(* Logix 5000 AddOnInstructionDefinition export Banner_S15S_TH_Param_v4; software revision 33.03 *)

TYPE Banner_Direct_Parameters_v4 :
STRUCT
   Master_Cycle_Time : INT;
   Min_Cycle_Time : INT;
   M_Sequence_Capability : INT;
   IO_Link_Version_ID : INT;
   Process_Data_Input_Length : INT;
   Process_Data_Output_Length : INT;
   Combined_Vendor_ID : DINT;   // IO-Link Vendor ID
   Vendor_ID1 : INT;
   Vendor_ID2 : INT;
   Combined_Device_ID : DINT;   // IO-Link Device ID
   Device_ID1 : INT;
   Device_ID2 : INT;
   Device_ID3 : INT;
END_STRUCT
END_TYPE

TYPE Banner_IOL_Port_v4 :   // UDT that has all of the data items necessary to communicate with a specific Port on a IO-Link Master
STRUCT
   Port_Controlled : INT;   // Each bit represents a port on an IO-Link Master. Set to 1 to tell AOI to control that port.
   Port_Activate : INT;   // Each bit represents a port on an IO-Link Master. When ON that port will process any commands in queue.
   Port_Read : INT;   // Each bit represents a port on an IO-Link Master. Used to determine when device AOI has requested a Read command.
   Port_Write : INT;   // Each bit represents a port on an IO-Link Master. Used to determine when device AOI has requested a Write command.
   Port_RW_Complete : INT;   // Each bit represents a port on an IO-Link Master. Tells device AOI that Read or Write request has been completed.
   Port_Device_Read : INT;
   Data_Transfer : SINT[190];   // Array to transfer data from IO-Master to device AOIs.
END_STRUCT
END_TYPE

TYPE Banner_S15S_TH_Alarm_Configuration_v4 :
STRUCT
   Temp_Low_Threshold : REAL;
   Temp_High_Threshold : REAL;
   Relative_Humidity_Low_Threshold : REAL;
   Relative_Humidity_High_Threshold : REAL;
   Dew_Point_Low_Threshold : REAL;
   Dew_Point_High_Threshold : REAL;
   Temp_On_Delay : REAL;
   Temp_Off_Delay : REAL;
   Relative_Humidity_On_Delay : REAL;
   Relative_Humidity_Off_Delay : REAL;
   Dew_Point_On_Delay : REAL;
   Dew_Point_Off_Delay : REAL;
END_STRUCT
END_TYPE

TYPE Banner_S15S_TH_Alarm_Counters_v4 :
STRUCT
   Temp_Low_Counter : DINT;
   Temp_High_Counter : DINT;
   Relative_Humidity_Low_Counter : DINT;
   Relative_Humidity_High_Counter : DINT;
   Dew_Point_Low_Counter : DINT;
   Dew_Point_High_Counter : DINT;
END_STRUCT
END_TYPE

TYPE Banner_S15S_TH_RD_v4 :   // UDT that stores the Read Data for a S15S-TH-KQ.
STRUCT
   Direct : Banner_Direct_Parameters_v4;
   Serial_Number : STRING;
   All_Time_Run_Time : DINT;   // 0 to 2 Billion. 1/4 hr increments.
END_STRUCT
END_TYPE

TYPE Banner_S15S_TH_v4 :   // All of the parameters for a S15S-TH-KQ.
STRUCT
   Initial_Global_Read : BOOL;   // Determines if all of the IO-Link data has been read into the PLC yet
   Command : INT;   // Value placed in here will activate a read or write to a specifc IO-Link Index
   Read : Banner_S15S_TH_RD_v4;   // Read Only Data
   Write : Banner_S15S_TH_WD_v4;   // Write Data
   Reset : BOOL;   // Resets AOI. This will force a complete parameter read of the sensor.
END_STRUCT
END_TYPE

TYPE Banner_S15S_TH_WD_v4 :   // UDT that stores the Write Data for a S15S-TH-KQ.
STRUCT
   System_Command : INT;   // See IODD file for list of commands that can be activated via the System Command interface
   Parameter_Access_Lock : SINT;   // Write access to all parameters is prohibited while value is 1. Only this parameter can be adjusted when value is 1.
   Data_Storage_Lock : SINT;   // Automatic data storage is disabled when this value is equal to 1. Read access is not affected.
   Local_Parameterization_Lock : SINT;   // Parameterization via local control elements on device is disabled.
   Local_User_Interface_Lock : SINT;   // Operation of local user interface is disabled.
   Resettable_Run_Time_Counter : DINT;   // 0 to 2 Billion. 1/4 hr increments.
   Alarm_Config : Banner_S15S_TH_Alarm_Configuration_v4;
   Alarm_Counters : Banner_S15S_TH_Alarm_Counters_v4;
   Process_Data_Mode : INT;   // 1=Smart Sensor Profile, Fahrenheit, 2=Smart Sensor Profile, Celsius, 3=Floating Point, Fahrenheit, 4=Floating Point, Celsius
   Output_Config : INT;   // 0=BannerBus,1=Discrete Output
END_STRUCT
END_TYPE

ADD_ON_INSTRUCTION Banner_S15S_TH_Float_In_v4   (* revision 4.0 *)
// AOI the orientates the bytes for a floating point value.
VAR_IN_OUT
   Float : REAL; {required}
END_VAR
VAR_INPUT
   Sint0 : SINT; {required}
   Sint1 : SINT; {required}
   Sint2 : SINT; {required}
   Sint3 : SINT; {required}
END_VAR
VAR
   Temp_Byte : SINT[4]; {access None}
END_VAR

ROUTINE Logic   (* ladder *)
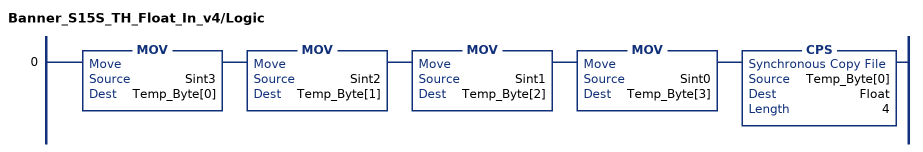
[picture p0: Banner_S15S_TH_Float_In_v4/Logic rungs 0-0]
   0: MOV(Sint3,Temp_Byte[0])MOV(Sint2,Temp_Byte[1])MOV(Sint1,Temp_Byte[2])MOV(Sint0,Temp_Byte[3])CPS(Temp_Byte[0],Float,4);
END_ROUTINE
END_ADD_ON_INSTRUCTION

ADD_ON_INSTRUCTION Banner_S15S_TH_Float_Out_v4   (* revision 4.0 *)
// AOI the orientates the bytes for a floating point value.
VAR_INPUT
   Float : REAL; {required}
END_VAR
VAR_IN_OUT
   Sint0 : SINT; {required}
   Sint1 : SINT; {required}
   Sint2 : SINT; {required}
   Sint3 : SINT; {required}
END_VAR
VAR
   Temp_Byte : SINT[4]; {access None}
END_VAR

ROUTINE Logic   (* ladder *)
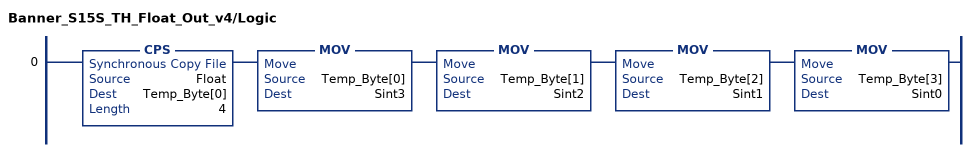
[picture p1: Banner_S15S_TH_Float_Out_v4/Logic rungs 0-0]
   0: CPS(Float,Temp_Byte[0],4)MOV(Temp_Byte[0],Sint3)MOV(Temp_Byte[1],Sint2)MOV(Temp_Byte[2],Sint1)MOV(Temp_Byte[3],Sint0);
END_ROUTINE
END_ADD_ON_INSTRUCTION

ADD_ON_INSTRUCTION Banner_S15S_TH_Param_v4   (* revision 4.0, vendor Banner Engineering *)
// AOI to read and write parameter data to an IO-Link S15S-TH-KQ.
VAR_IN_OUT
   S15STH : Banner_S15S_TH_v4; {required}
   Port_Data : Banner_IOL_Port_v4; {required}
END_VAR
VAR_INPUT
   Port : DINT; {required}
END_VAR
VAR
   Local_Control : DINT; {access None}
   Global_Read_Command_Value : INT; {access None}
   Global_Write_Command_Value : INT; {access None}
   Command_Being_Processed : BOOL; {access None}
   Update_Archive : BOOL; {access None}
   Index_Write_Inprocess : INT; {access None}
   Index_Write_Control : INT; {access None}
   Inprocess_Index : DINT; {access None}
   AOI_Out_Status : Banner_S15S_TH_Float_Out_v4[12]; {access None}
   AOI_In_Status : Banner_S15S_TH_Float_In_v4[12]; {access None}
END_VAR

ROUTINE Logic   (* ladder *)
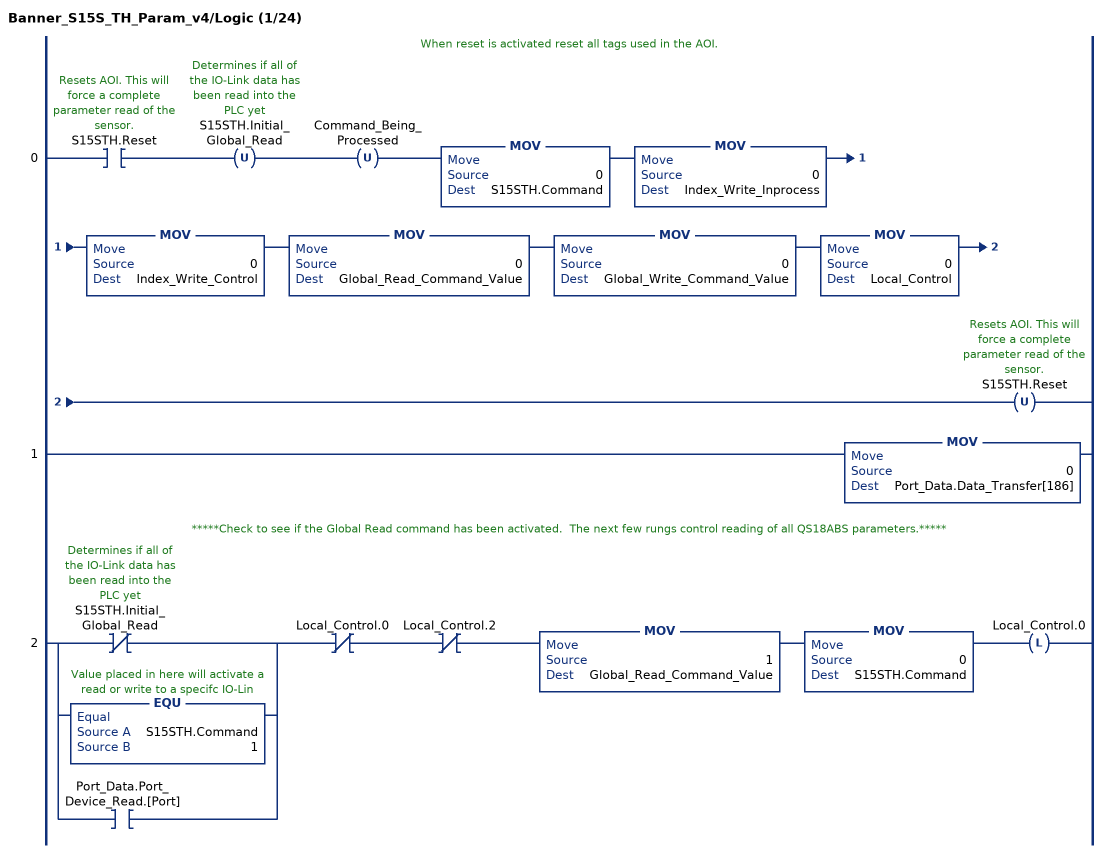
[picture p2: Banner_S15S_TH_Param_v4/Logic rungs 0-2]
   // When reset is activated reset all tags used in the AOI.
   0: XIC(S15STH.Reset)OTU(S15STH.Initial_Global_Read)OTU(Command_Being_Processed)MOV(0,S15STH.Command)MOV(0,Index_Write_Inprocess)MOV(0,Index_Write_Control)MOV(0,Global_Read_Command_Value)MOV(0,Global_Write_Command_Value)MOV(0,Local_Control)OTU(S15STH.Reset);
   1: MOV(0,Port_Data.Data_Transfer[186]);
   // *****Check to see if the Global Read command has been activated.  The next few rungs control reading of all QS18ABS parameters.*****
   2: [XIO(S15STH.Initial_Global_Read) ,EQU(S15STH.Command,1) ,XIC(Port_Data.Port_Device_Read.[Port]) ]XIO(Local_Control.0)XIO(Local_Control.2)MOV(1,Global_Read_Command_Value)MOV(0,S15STH.Command)OTL(Local_Control.0);
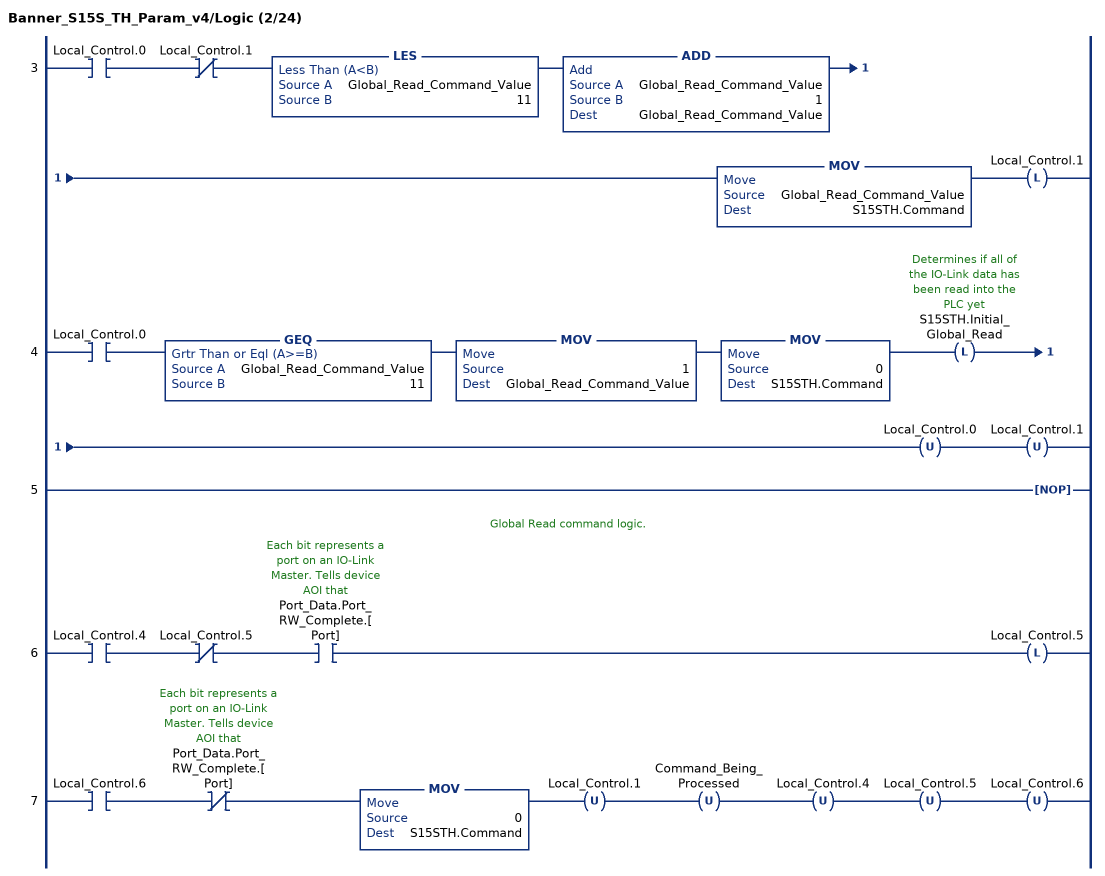
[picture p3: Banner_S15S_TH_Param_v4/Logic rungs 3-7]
   3: XIC(Local_Control.0)XIO(Local_Control.1)LES(Global_Read_Command_Value,11)ADD(Global_Read_Command_Value,1,Global_Read_Command_Value)MOV(Global_Read_Command_Value,S15STH.Command)OTL(Local_Control.1);
   4: XIC(Local_Control.0)GEQ(Global_Read_Command_Value,11)MOV(1,Global_Read_Command_Value)MOV(0,S15STH.Command)OTL(S15STH.Initial_Global_Read)OTU(Local_Control.0)OTU(Local_Control.1);
   5: NOP();
   // Global Read command logic.
   6: XIC(Local_Control.4)XIO(Local_Control.5)XIC(Port_Data.Port_RW_Complete.[Port])OTL(Local_Control.5);
   7: XIC(Local_Control.6)XIO(Port_Data.Port_RW_Complete.[Port])MOV(0,S15STH.Command)OTU(Local_Control.1)OTU(Command_Being_Processed)OTU(Local_Control.4)OTU(Local_Control.5)OTU(Local_Control.6);
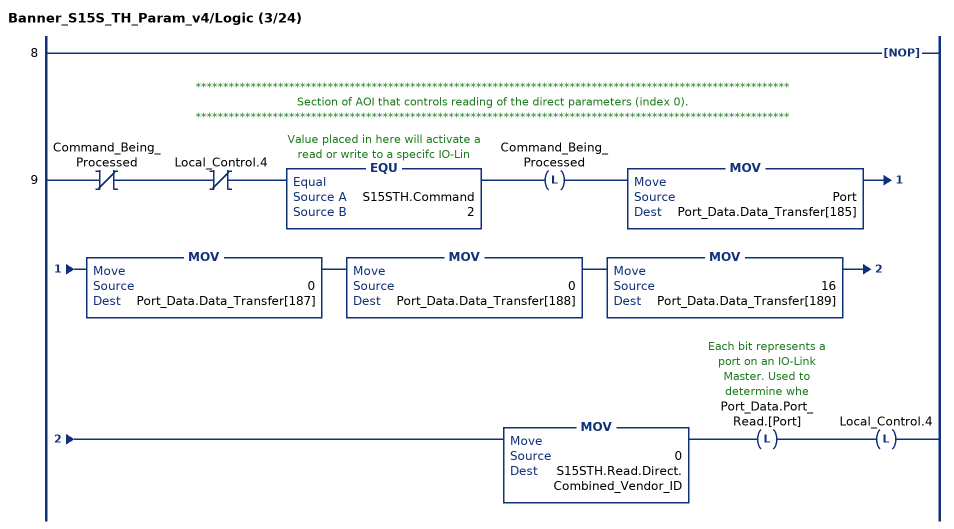
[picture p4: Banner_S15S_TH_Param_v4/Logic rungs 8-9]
   8: NOP();
   // ************************************************************************************************************
   // Section of AOI that controls reading of the direct parameters (index 0).
   // ************************************************************************************************************
   9: XIO(Command_Being_Processed)XIO(Local_Control.4)EQU(S15STH.Command,2)OTL(Command_Being_Processed)MOV(Port,Port_Data.Data_Transfer[185])MOV(0,Port_Data.Data_Transfer[187])MOV(0,Port_Data.Data_Transfer[188])MOV(16,Port_Data.Data_Transfer[189])MOV(0,S15STH.Read.Direct.Combined_Vendor_ID)OTL(Port_Data.Port_Read.[Port])OTL(Local_Control.4);
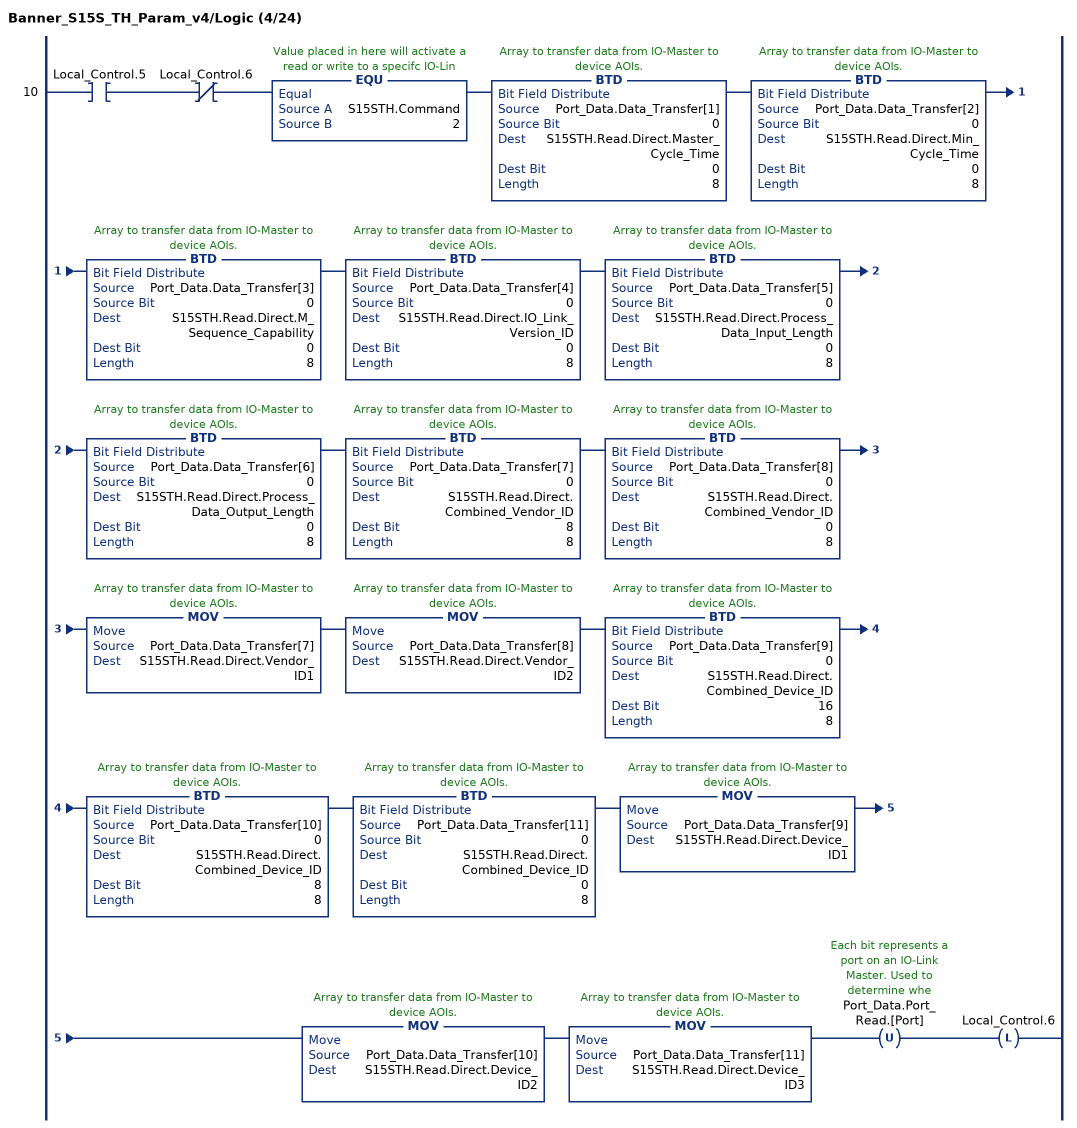
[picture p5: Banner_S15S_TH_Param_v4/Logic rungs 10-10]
   10: XIC(Local_Control.5)XIO(Local_Control.6)EQU(S15STH.Command,2)BTD(Port_Data.Data_Transfer[1],0,S15STH.Read.Direct.Master_Cycle_Time,0,8)BTD(Port_Data.Data_Transfer[2],0,S15STH.Read.Direct.Min_Cycle_Time,0,8)BTD(Port_Data.Data_Transfer[3],0,S15STH.Read.Direct.M_Sequence_Capability,0,8)BTD(Port_Data.Data_Transfer[4],0,S15STH.Read.Direct.IO_Link_Version_ID,0,8)BTD(Port_Data.Data_Transfer[5],0,S15STH.Read.Direct.Process_Data_Input_Length,0,8)BTD(Port_Data.Data_Transfer[6],0,S15STH.Read.Direct.Process_Data_Output_Length,0,8)BTD(Port_Data.Data_Transfer[7],0,S15STH.Read.Direct.Combined_Vendor_ID,8,8)BTD(Port_Data.Data_Transfer[8],0,S15STH.Read.Direct.Combined_Vendor_ID,0,8)MOV(Port_Data.Data_Transfer[7],S15STH.Read.Direct.Vendor_ID1)MOV(Port_Data.Data_Transfer[8],S15STH.Read.Direct.Vendor_ID2)BTD(Port_Data.Data_Transfer[9],0,S15STH.Read.Direct.Combined_Device_ID,16,8)BTD(Port_Data.Data_Transfer[10],0,S15STH.Read.Direct.Combined_Device_ID,8,8)BTD(Port_Data.Data_Transfer[11],0,S15STH.Read.Direct.Combined_Device_ID,0,8)MOV(Port_Data.Data_Transfer[9],S15STH.Read.Direct.Device_ID1)MOV(Port_Data.Data_Transfer[10],S15STH.Read.Direct.Device_ID2)MOV(Port_Data.Data_Transfer[11],S15STH.Read.Direct.Device_ID3)OTU(Port_Data.Port_Read.[Port])OTL(Local_Control.6);
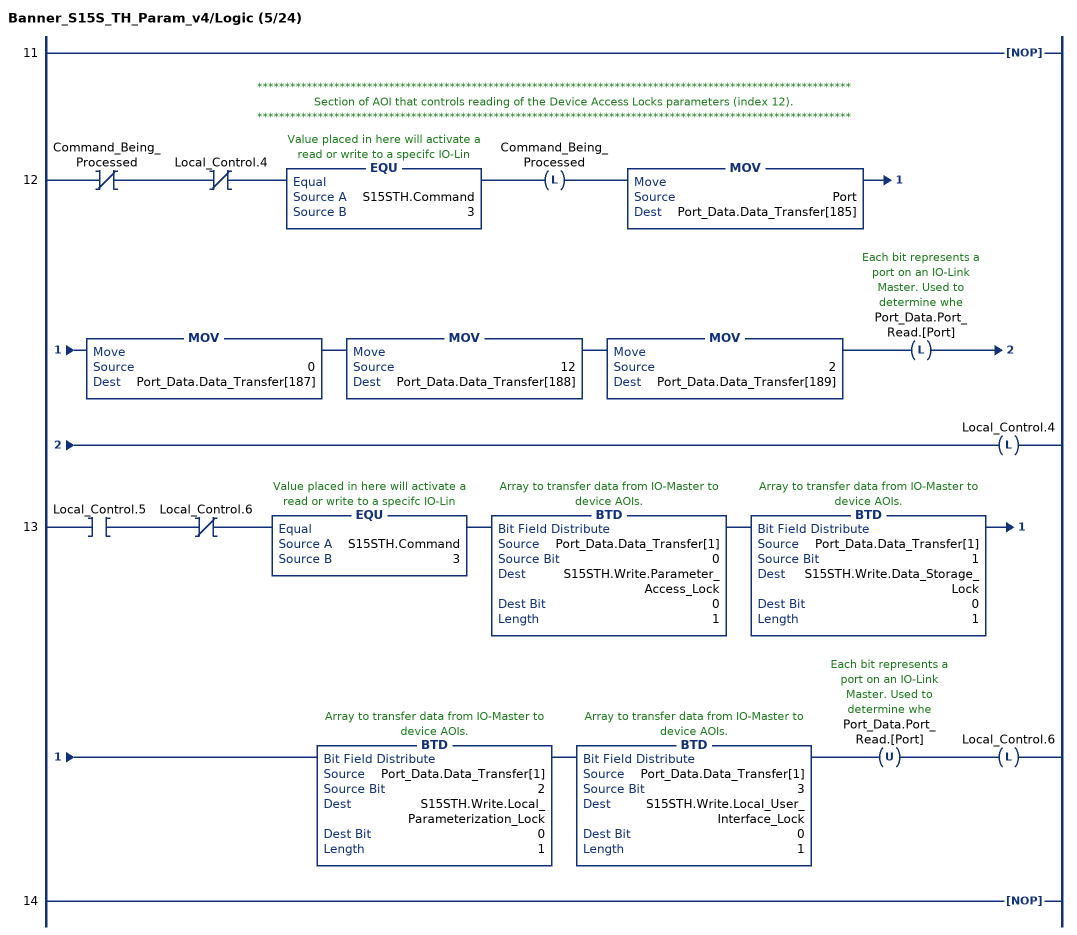
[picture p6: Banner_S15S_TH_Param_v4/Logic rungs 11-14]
   11: NOP();
   // ************************************************************************************************************
   // Section of AOI that controls reading of the Device Access Locks parameters (index 12).
   // ************************************************************************************************************
   12: XIO(Command_Being_Processed)XIO(Local_Control.4)EQU(S15STH.Command,3)OTL(Command_Being_Processed)MOV(Port,Port_Data.Data_Transfer[185])MOV(0,Port_Data.Data_Transfer[187])MOV(12,Port_Data.Data_Transfer[188])MOV(2,Port_Data.Data_Transfer[189])OTL(Port_Data.Port_Read.[Port])OTL(Local_Control.4);
   13: XIC(Local_Control.5)XIO(Local_Control.6)EQU(S15STH.Command,3)BTD(Port_Data.Data_Transfer[1],0,S15STH.Write.Parameter_Access_Lock,0,1)BTD(Port_Data.Data_Transfer[1],1,S15STH.Write.Data_Storage_Lock,0,1)BTD(Port_Data.Data_Transfer[1],2,S15STH.Write.Local_Parameterization_Lock,0,1)BTD(Port_Data.Data_Transfer[1],3,S15STH.Write.Local_User_Interface_Lock,0,1)OTU(Port_Data.Port_Read.[Port])OTL(Local_Control.6);
   14: NOP();
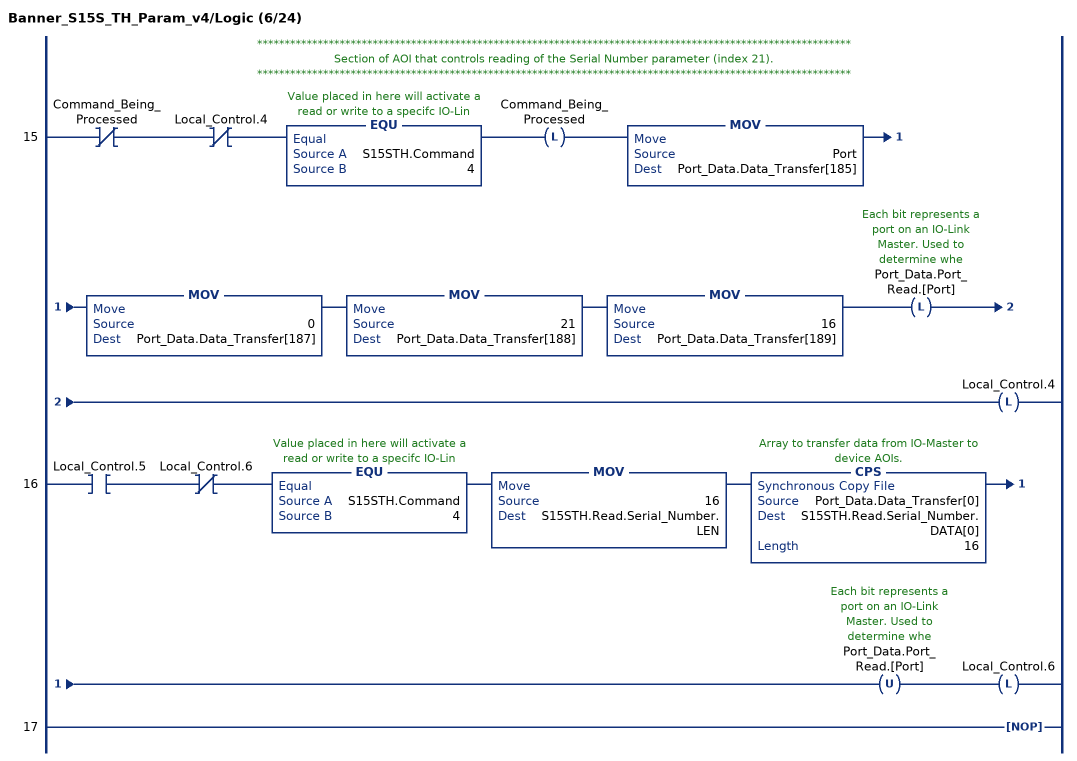
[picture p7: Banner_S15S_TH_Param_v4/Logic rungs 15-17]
   // ************************************************************************************************************
   // Section of AOI that controls reading of the Serial Number parameter (index 21).
   // ************************************************************************************************************
   15: XIO(Command_Being_Processed)XIO(Local_Control.4)EQU(S15STH.Command,4)OTL(Command_Being_Processed)MOV(Port,Port_Data.Data_Transfer[185])MOV(0,Port_Data.Data_Transfer[187])MOV(21,Port_Data.Data_Transfer[188])MOV(16,Port_Data.Data_Transfer[189])OTL(Port_Data.Port_Read.[Port])OTL(Local_Control.4);
   16: XIC(Local_Control.5)XIO(Local_Control.6)EQU(S15STH.Command,4)MOV(16,S15STH.Read.Serial_Number.LEN)CPS(Port_Data.Data_Transfer[0],S15STH.Read.Serial_Number.DATA[0],16)OTU(Port_Data.Port_Read.[Port])OTL(Local_Control.6);
   17: NOP();
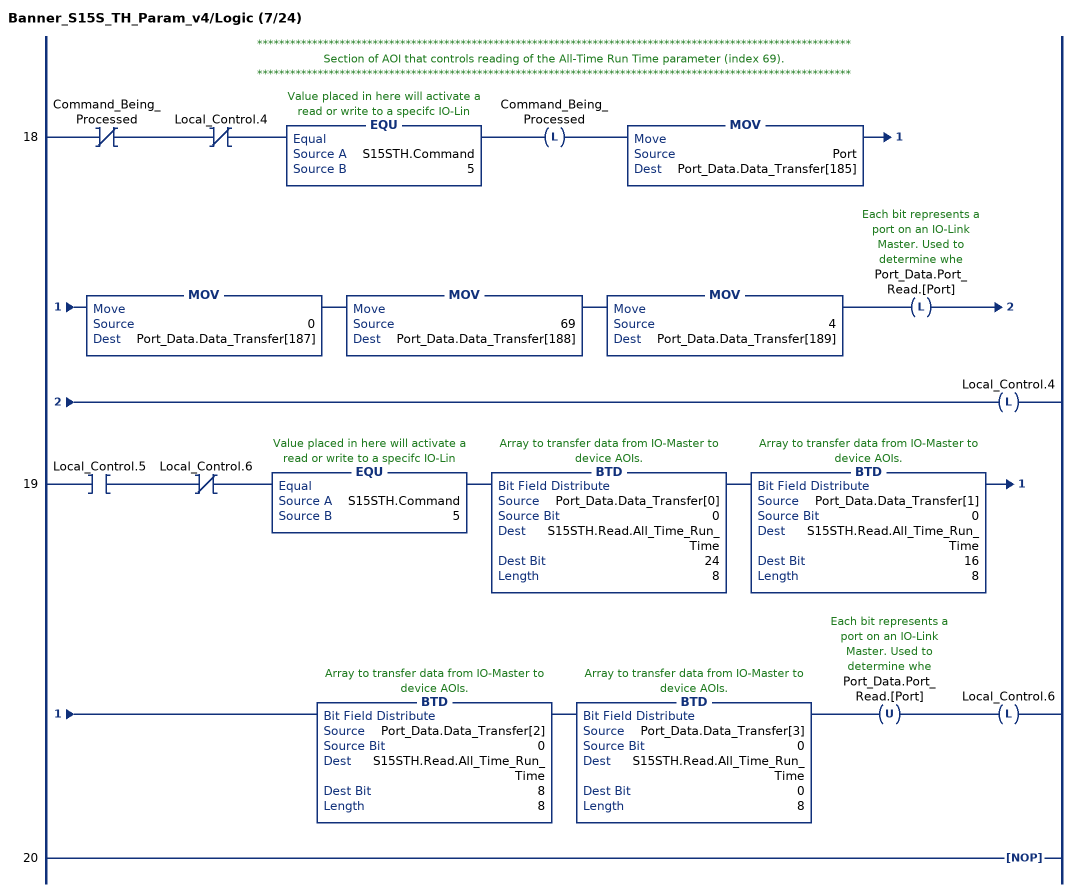
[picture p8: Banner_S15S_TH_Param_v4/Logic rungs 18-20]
   // ************************************************************************************************************
   // Section of AOI that controls reading of the All-Time Run Time parameter (index 69).
   // ************************************************************************************************************
   18: XIO(Command_Being_Processed)XIO(Local_Control.4)EQU(S15STH.Command,5)OTL(Command_Being_Processed)MOV(Port,Port_Data.Data_Transfer[185])MOV(0,Port_Data.Data_Transfer[187])MOV(69,Port_Data.Data_Transfer[188])MOV(4,Port_Data.Data_Transfer[189])OTL(Port_Data.Port_Read.[Port])OTL(Local_Control.4);
   19: XIC(Local_Control.5)XIO(Local_Control.6)EQU(S15STH.Command,5)BTD(Port_Data.Data_Transfer[0],0,S15STH.Read.All_Time_Run_Time,24,8)BTD(Port_Data.Data_Transfer[1],0,S15STH.Read.All_Time_Run_Time,16,8)BTD(Port_Data.Data_Transfer[2],0,S15STH.Read.All_Time_Run_Time,8,8)BTD(Port_Data.Data_Transfer[3],0,S15STH.Read.All_Time_Run_Time,0,8)OTU(Port_Data.Port_Read.[Port])OTL(Local_Control.6);
   20: NOP();
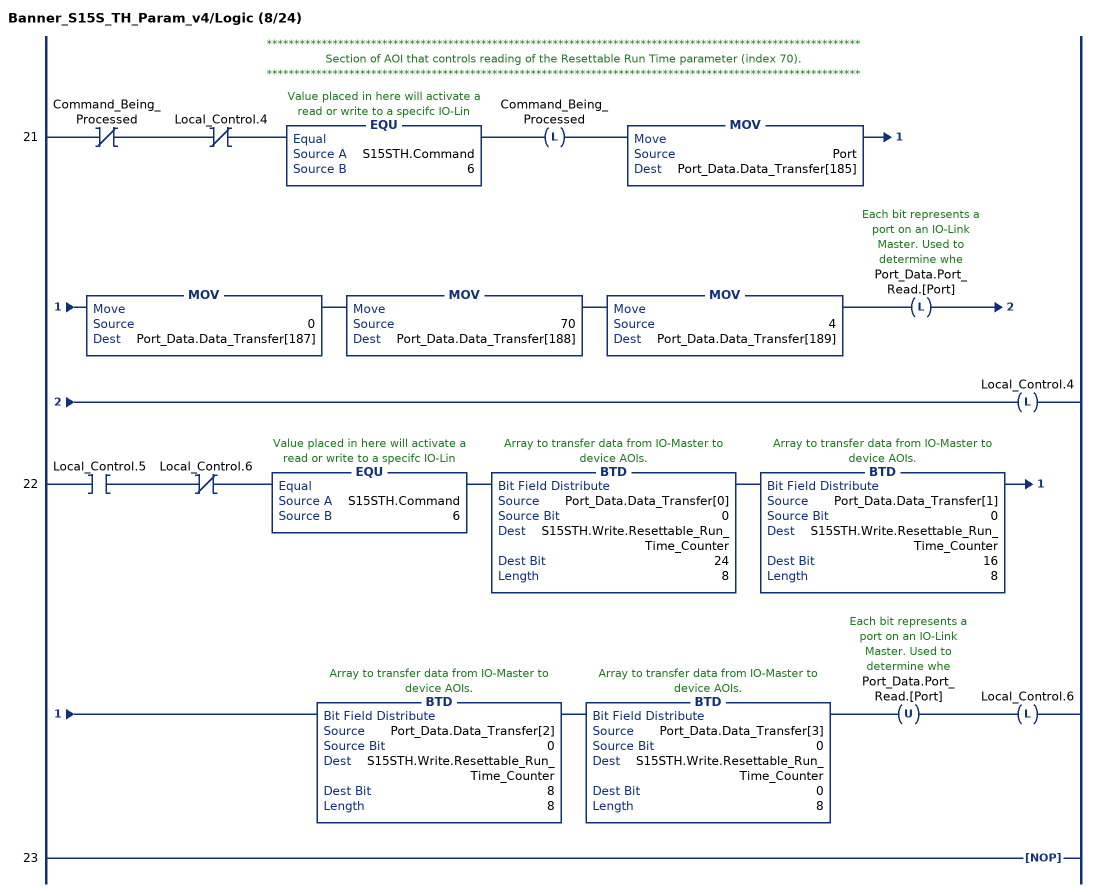
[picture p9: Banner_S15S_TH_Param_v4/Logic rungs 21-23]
   // ************************************************************************************************************
   // Section of AOI that controls reading of the Resettable Run Time parameter (index 70).
   // ************************************************************************************************************
   21: XIO(Command_Being_Processed)XIO(Local_Control.4)EQU(S15STH.Command,6)OTL(Command_Being_Processed)MOV(Port,Port_Data.Data_Transfer[185])MOV(0,Port_Data.Data_Transfer[187])MOV(70,Port_Data.Data_Transfer[188])MOV(4,Port_Data.Data_Transfer[189])OTL(Port_Data.Port_Read.[Port])OTL(Local_Control.4);
   22: XIC(Local_Control.5)XIO(Local_Control.6)EQU(S15STH.Command,6)BTD(Port_Data.Data_Transfer[0],0,S15STH.Write.Resettable_Run_Time_Counter,24,8)BTD(Port_Data.Data_Transfer[1],0,S15STH.Write.Resettable_Run_Time_Counter,16,8)BTD(Port_Data.Data_Transfer[2],0,S15STH.Write.Resettable_Run_Time_Counter,8,8)BTD(Port_Data.Data_Transfer[3],0,S15STH.Write.Resettable_Run_Time_Counter,0,8)OTU(Port_Data.Port_Read.[Port])OTL(Local_Control.6);
   23: NOP();
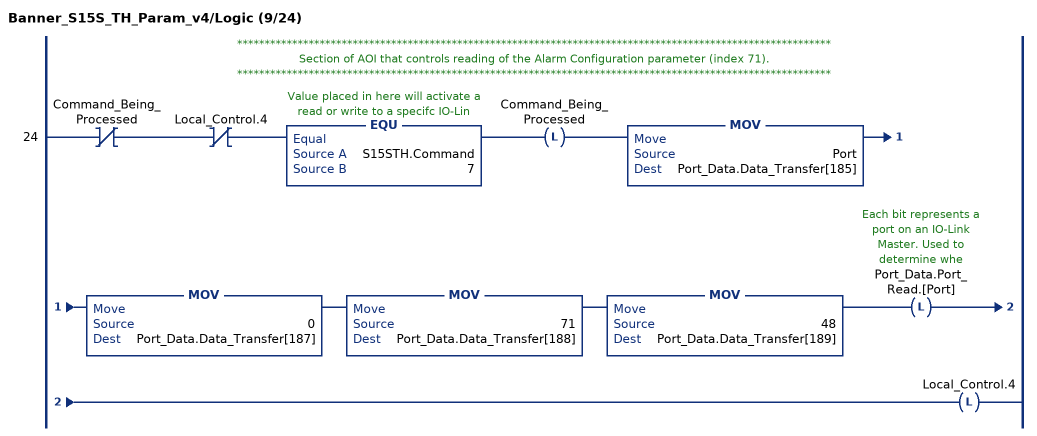
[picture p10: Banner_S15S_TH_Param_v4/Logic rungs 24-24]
   // ************************************************************************************************************
   // Section of AOI that controls reading of the Alarm Configuration parameter (index 71).
   // ************************************************************************************************************
   24: XIO(Command_Being_Processed)XIO(Local_Control.4)EQU(S15STH.Command,7)OTL(Command_Being_Processed)MOV(Port,Port_Data.Data_Transfer[185])MOV(0,Port_Data.Data_Transfer[187])MOV(71,Port_Data.Data_Transfer[188])MOV(48,Port_Data.Data_Transfer[189])OTL(Port_Data.Port_Read.[Port])OTL(Local_Control.4);
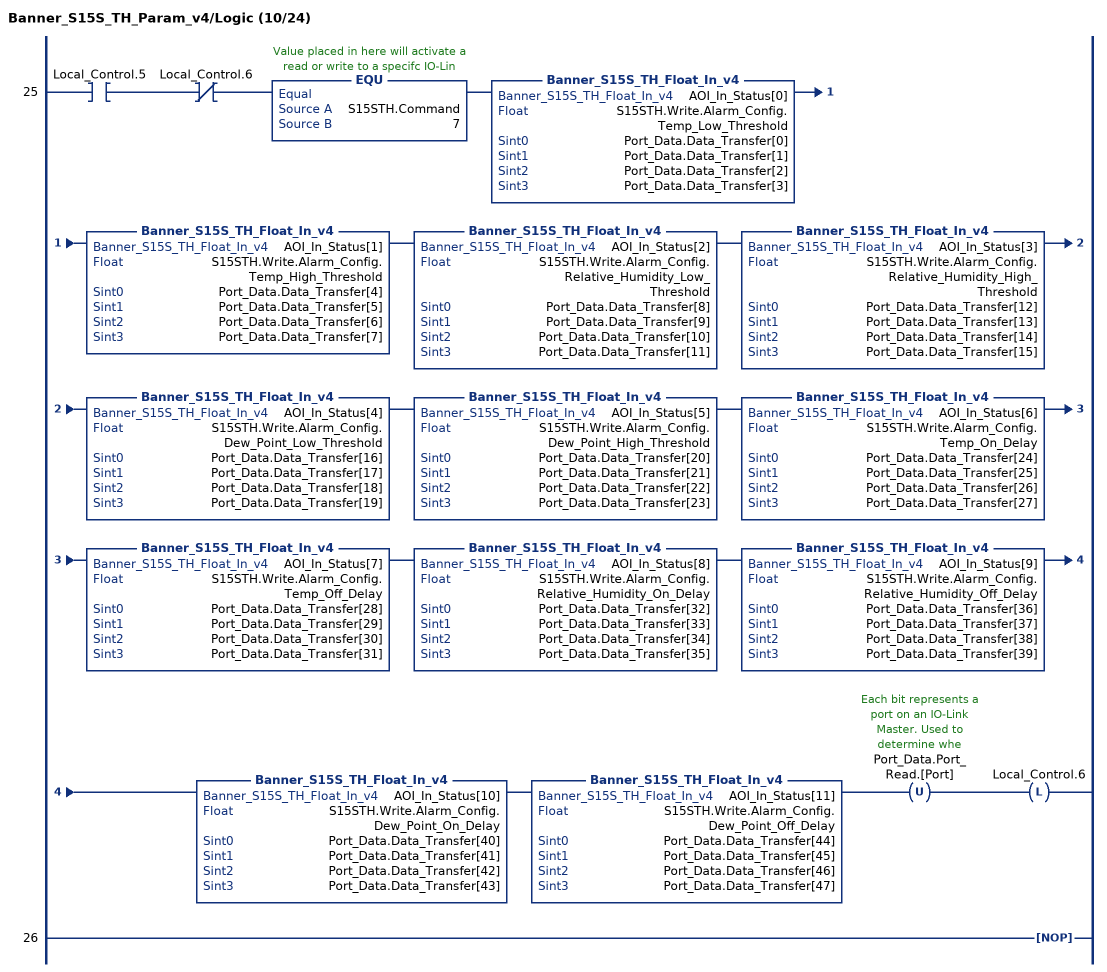
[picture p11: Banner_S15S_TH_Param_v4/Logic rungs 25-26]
   25: XIC(Local_Control.5)XIO(Local_Control.6)EQU(S15STH.Command,7)Banner_S15S_TH_Float_In_v4(AOI_In_Status[0],S15STH.Write.Alarm_Config.Temp_Low_Threshold,Port_Data.Data_Transfer[0],Port_Data.Data_Transfer[1],Port_Data.Data_Transfer[2],Port_Data.Data_Transfer[3])Banner_S15S_TH_Float_In_v4(AOI_In_Status[1],S15STH.Write.Alarm_Config.Temp_High_Threshold,Port_Data.Data_Transfer[4],Port_Data.Data_Transfer[5],Port_Data.Data_Transfer[6],Port_Data.Data_Transfer[7])Banner_S15S_TH_Float_In_v4(AOI_In_Status[2],S15STH.Write.Alarm_Config.Relative_Humidity_Low_Threshold,Port_Data.Data_Transfer[8],Port_Data.Data_Transfer[9],Port_Data.Data_Transfer[10],Port_Data.Data_Transfer[11])Banner_S15S_TH_Float_In_v4(AOI_In_Status[3],S15STH.Write.Alarm_Config.Relative_Humidity_High_Threshold,Port_Data.Data_Transfer[12],Port_Data.Data_Transfer[13],Port_Data.Data_Transfer[14],Port_Data.Data_Transfer[15])Banner_S15S_TH_Float_In_v4(AOI_In_Status[4],S15STH.Write.Alarm_Config.Dew_Point_Low_Threshold,Port_Data.Data_Transfer[16],Port_Data.Data_Transfer[17],Port_Data.Data_Transfer[18],Port_Data.Data_Transfer[19])Banner_S15S_TH_Float_In_v4(AOI_In_Status[5],S15STH.Write.Alarm_Config.Dew_Point_High_Threshold,Port_Data.Data_Transfer[20],Port_Data.Data_Transfer[21],Port_Data.Data_Transfer[22],Port_Data.Data_Transfer[23])Banner_S15S_TH_Float_In_v4(AOI_In_Status[6],S15STH.Write.Alarm_Config.Temp_On_Delay,Port_Data.Data_Transfer[24],Port_Data.Data_Transfer[25],Port_Data.Data_Transfer[26],Port_Data.Data_Transfer[27])Banner_S15S_TH_Float_In_v4(AOI_In_Status[7],S15STH.Write.Alarm_Config.Temp_Off_Delay,Port_Data.Data_Transfer[28],Port_Data.Data_Transfer[29],Port_Data.Data_Transfer[30],Port_Data.Data_Transfer[31])Banner_S15S_TH_Float_In_v4(AOI_In_Status[8],S15STH.Write.Alarm_Config.Relative_Humidity_On_Delay,Port_Data.Data_Transfer[32],Port_Data.Data_Transfer[33],Port_Data.Data_Transfer[34],Port_Data.Data_Transfer[35])Banner_S15S_TH_Float_In_v4(AOI_In_Status[9],S15STH.Write.Alarm_Config.Relative_Humidity_Off_Delay,Port_Data.Data_Transfer[36],Port_Data.Data_Transfer[37],Port_Data.Data_Transfer[38],Port_Data.Data_Transfer[39])Banner_S15S_TH_Float_In_v4(AOI_In_Status[10],S15STH.Write.Alarm_Config.Dew_Point_On_Delay,Port_Data.Data_Transfer[40],Port_Data.Data_Transfer[41],Port_Data.Data_Transfer[42],Port_Data.Data_Transfer[43])Banner_S15S_TH_Float_In_v4(AOI_In_Status[11],S15STH.Write.Alarm_Config.Dew_Point_Off_Delay,Port_Data.Data_Transfer[44],Port_Data.Data_Transfer[45],Port_Data.Data_Transfer[46],Port_Data.Data_Transfer[47])OTU(Port_Data.Port_Read.[Port])OTL(Local_Control.6);
   26: NOP();
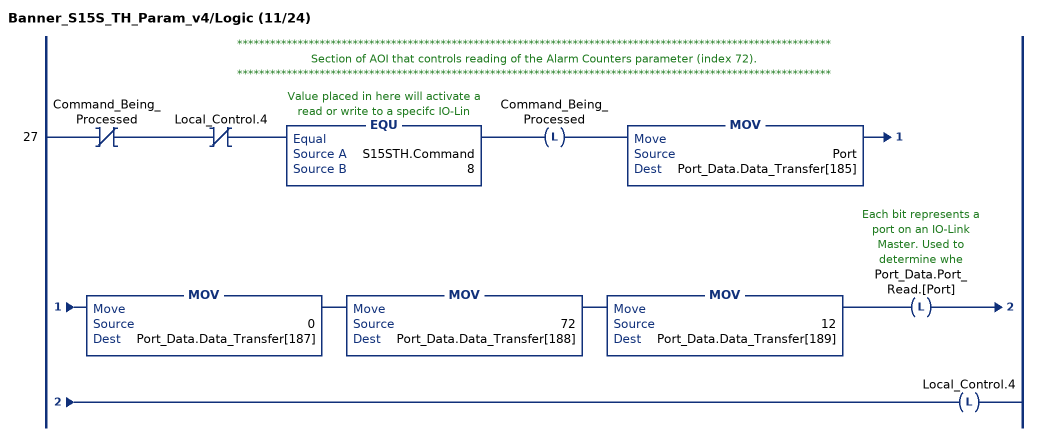
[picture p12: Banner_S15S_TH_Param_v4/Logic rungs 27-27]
   // ************************************************************************************************************
   // Section of AOI that controls reading of the Alarm Counters parameter (index 72).
   // ************************************************************************************************************
   27: XIO(Command_Being_Processed)XIO(Local_Control.4)EQU(S15STH.Command,8)OTL(Command_Being_Processed)MOV(Port,Port_Data.Data_Transfer[185])MOV(0,Port_Data.Data_Transfer[187])MOV(72,Port_Data.Data_Transfer[188])MOV(12,Port_Data.Data_Transfer[189])OTL(Port_Data.Port_Read.[Port])OTL(Local_Control.4);
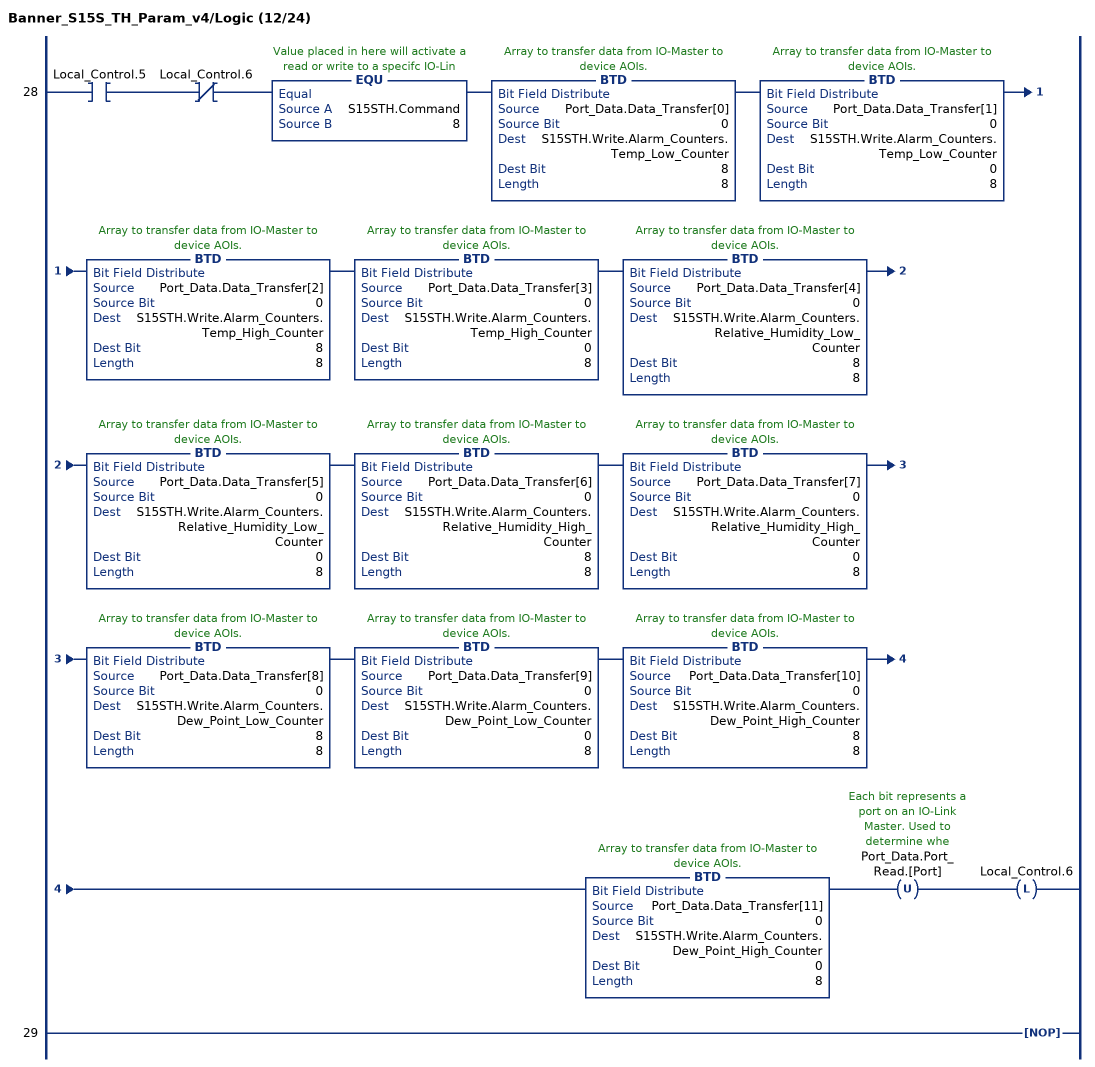
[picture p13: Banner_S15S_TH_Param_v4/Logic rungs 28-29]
   28: XIC(Local_Control.5)XIO(Local_Control.6)EQU(S15STH.Command,8)BTD(Port_Data.Data_Transfer[0],0,S15STH.Write.Alarm_Counters.Temp_Low_Counter,8,8)BTD(Port_Data.Data_Transfer[1],0,S15STH.Write.Alarm_Counters.Temp_Low_Counter,0,8)BTD(Port_Data.Data_Transfer[2],0,S15STH.Write.Alarm_Counters.Temp_High_Counter,8,8)BTD(Port_Data.Data_Transfer[3],0,S15STH.Write.Alarm_Counters.Temp_High_Counter,0,8)BTD(Port_Data.Data_Transfer[4],0,S15STH.Write.Alarm_Counters.Relative_Humidity_Low_Counter,8,8)BTD(Port_Data.Data_Transfer[5],0,S15STH.Write.Alarm_Counters.Relative_Humidity_Low_Counter,0,8)BTD(Port_Data.Data_Transfer[6],0,S15STH.Write.Alarm_Counters.Relative_Humidity_High_Counter,8,8)BTD(Port_Data.Data_Transfer[7],0,S15STH.Write.Alarm_Counters.Relative_Humidity_High_Counter,0,8)BTD(Port_Data.Data_Transfer[8],0,S15STH.Write.Alarm_Counters.Dew_Point_Low_Counter,8,8)BTD(Port_Data.Data_Transfer[9],0,S15STH.Write.Alarm_Counters.Dew_Point_Low_Counter,0,8)BTD(Port_Data.Data_Transfer[10],0,S15STH.Write.Alarm_Counters.Dew_Point_High_Counter,8,8)BTD(Port_Data.Data_Transfer[11],0,S15STH.Write.Alarm_Counters.Dew_Point_High_Counter,0,8)OTU(Port_Data.Port_Read.[Port])OTL(Local_Control.6);
   29: NOP();
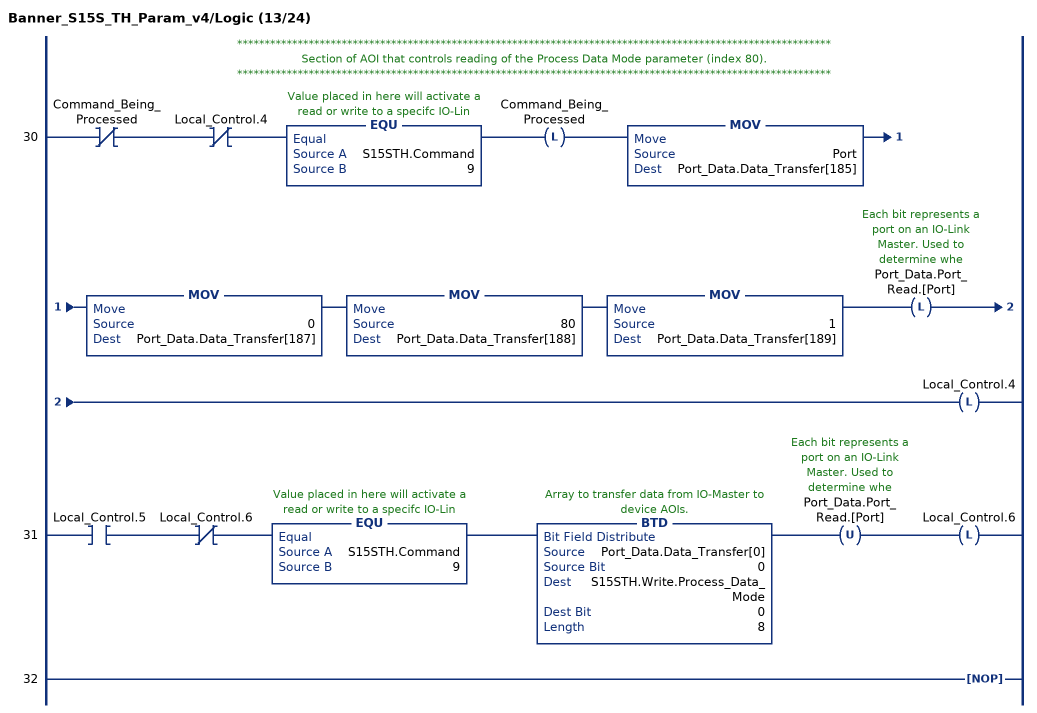
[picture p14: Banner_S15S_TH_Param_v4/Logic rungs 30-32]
   // ************************************************************************************************************
   // Section of AOI that controls reading of the Process Data Mode parameter (index 80).
   // ************************************************************************************************************
   30: XIO(Command_Being_Processed)XIO(Local_Control.4)EQU(S15STH.Command,9)OTL(Command_Being_Processed)MOV(Port,Port_Data.Data_Transfer[185])MOV(0,Port_Data.Data_Transfer[187])MOV(80,Port_Data.Data_Transfer[188])MOV(1,Port_Data.Data_Transfer[189])OTL(Port_Data.Port_Read.[Port])OTL(Local_Control.4);
   31: XIC(Local_Control.5)XIO(Local_Control.6)EQU(S15STH.Command,9)BTD(Port_Data.Data_Transfer[0],0,S15STH.Write.Process_Data_Mode,0,8)OTU(Port_Data.Port_Read.[Port])OTL(Local_Control.6);
   32: NOP();
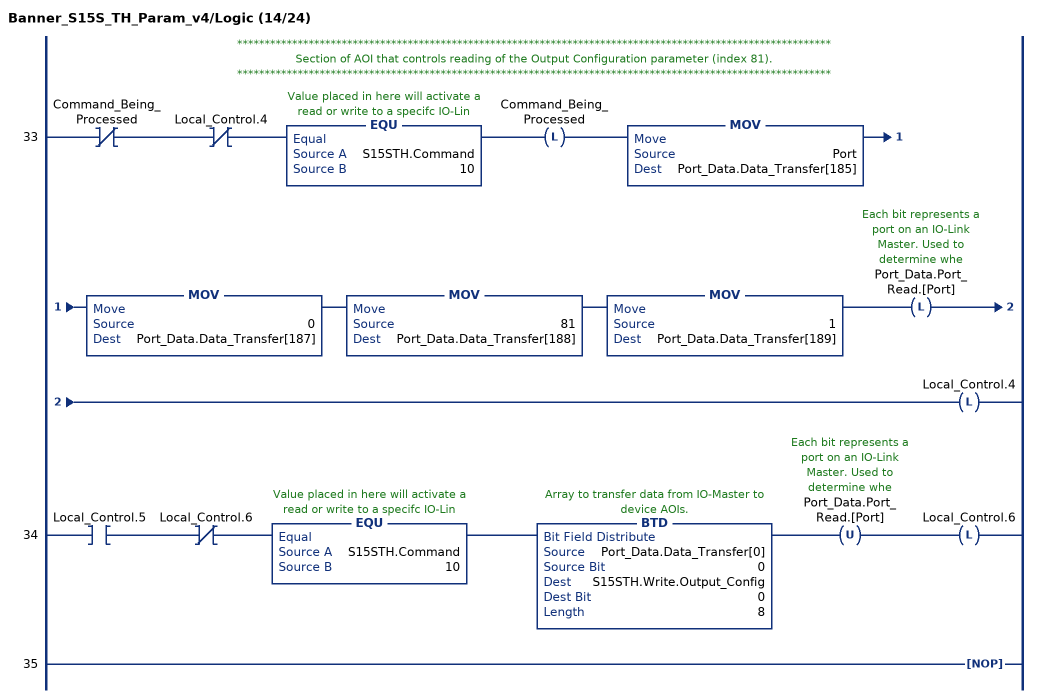
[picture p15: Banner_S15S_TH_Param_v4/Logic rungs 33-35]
   // ************************************************************************************************************
   // Section of AOI that controls reading of the Output Configuration parameter (index 81).
   // ************************************************************************************************************
   33: XIO(Command_Being_Processed)XIO(Local_Control.4)EQU(S15STH.Command,10)OTL(Command_Being_Processed)MOV(Port,Port_Data.Data_Transfer[185])MOV(0,Port_Data.Data_Transfer[187])MOV(81,Port_Data.Data_Transfer[188])MOV(1,Port_Data.Data_Transfer[189])OTL(Port_Data.Port_Read.[Port])OTL(Local_Control.4);
   34: XIC(Local_Control.5)XIO(Local_Control.6)EQU(S15STH.Command,10)BTD(Port_Data.Data_Transfer[0],0,S15STH.Write.Output_Config,0,8)OTU(Port_Data.Port_Read.[Port])OTL(Local_Control.6);
   35: NOP();
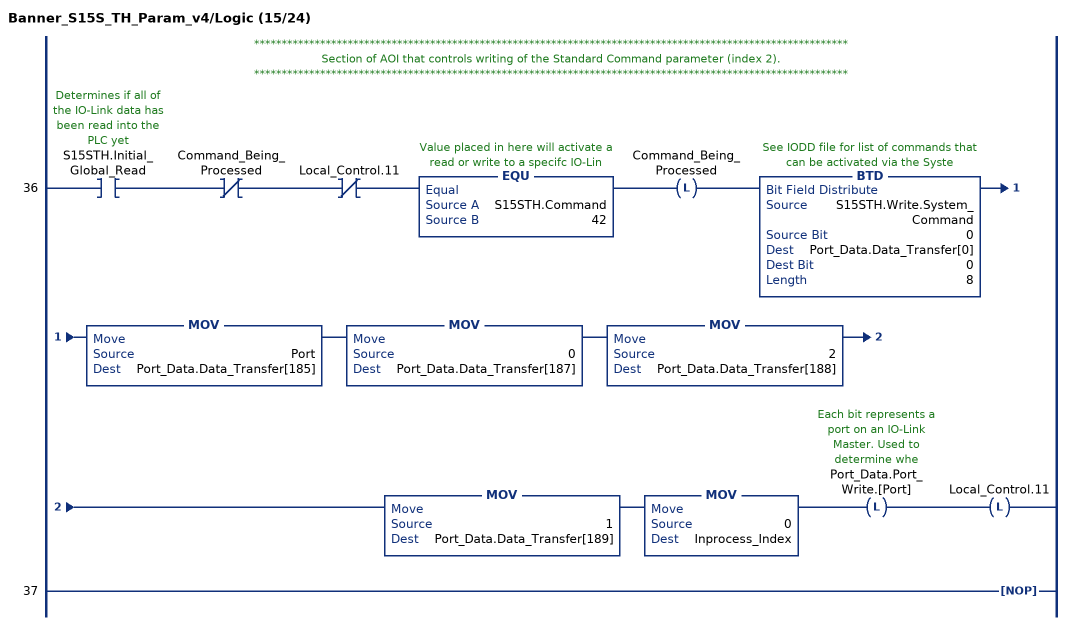
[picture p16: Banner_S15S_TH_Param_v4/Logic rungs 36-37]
   // ************************************************************************************************************
   // Section of AOI that controls writing of the Standard Command parameter (index 2).
   // ************************************************************************************************************
   36: XIC(S15STH.Initial_Global_Read)XIO(Command_Being_Processed)XIO(Local_Control.11)EQU(S15STH.Command,42)OTL(Command_Being_Processed)BTD(S15STH.Write.System_Command,0,Port_Data.Data_Transfer[0],0,8)MOV(Port,Port_Data.Data_Transfer[185])MOV(0,Port_Data.Data_Transfer[187])MOV(2,Port_Data.Data_Transfer[188])MOV(1,Port_Data.Data_Transfer[189])MOV(0,Inprocess_Index)OTL(Port_Data.Port_Write.[Port])OTL(Local_Control.11);
   37: NOP();
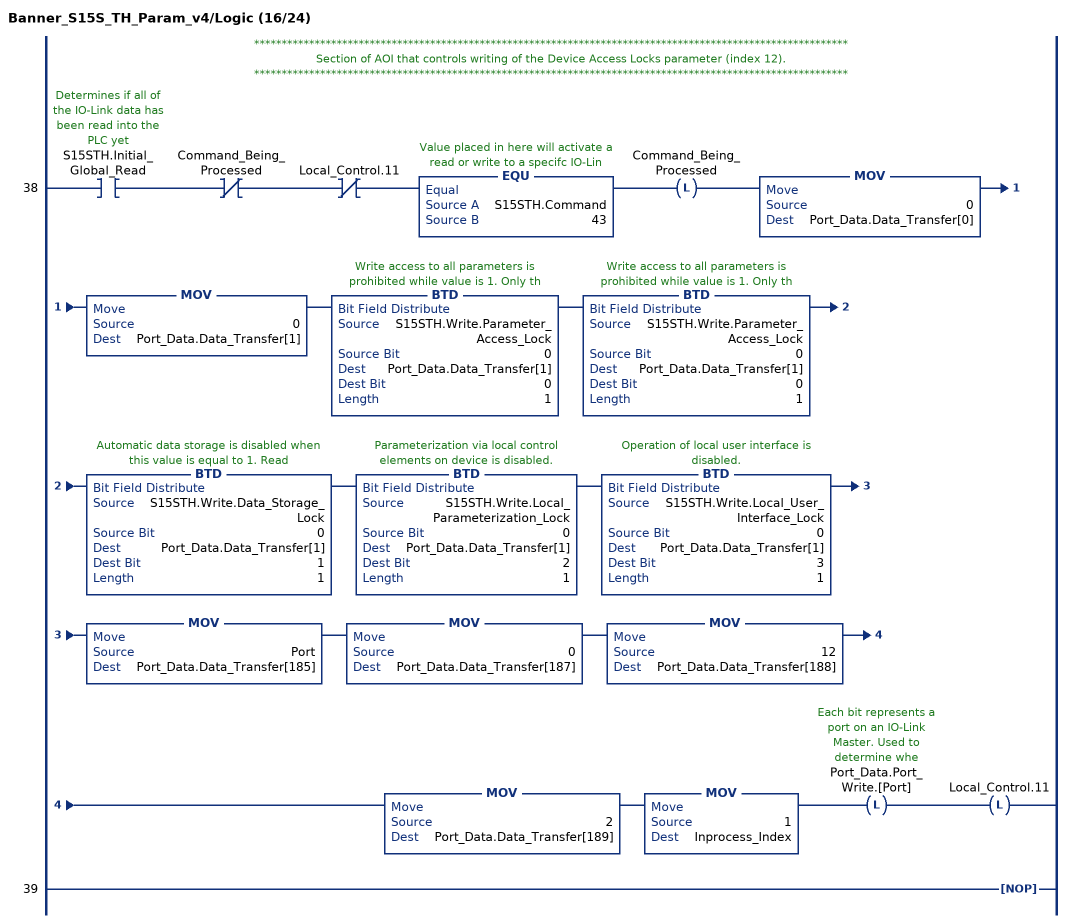
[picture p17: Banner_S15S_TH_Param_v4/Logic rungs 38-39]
   // ************************************************************************************************************
   // Section of AOI that controls writing of the Device Access Locks parameter (index 12).
   // ************************************************************************************************************
   38: XIC(S15STH.Initial_Global_Read)XIO(Command_Being_Processed)XIO(Local_Control.11)EQU(S15STH.Command,43)OTL(Command_Being_Processed)MOV(0,Port_Data.Data_Transfer[0])MOV(0,Port_Data.Data_Transfer[1])BTD(S15STH.Write.Parameter_Access_Lock,0,Port_Data.Data_Transfer[1],0,1)BTD(S15STH.Write.Parameter_Access_Lock,0,Port_Data.Data_Transfer[1],0,1)BTD(S15STH.Write.Data_Storage_Lock,0,Port_Data.Data_Transfer[1],1,1)BTD(S15STH.Write.Local_Parameterization_Lock,0,Port_Data.Data_Transfer[1],2,1)BTD(S15STH.Write.Local_User_Interface_Lock,0,Port_Data.Data_Transfer[1],3,1)MOV(Port,Port_Data.Data_Transfer[185])MOV(0,Port_Data.Data_Transfer[187])MOV(12,Port_Data.Data_Transfer[188])MOV(2,Port_Data.Data_Transfer[189])MOV(1,Inprocess_Index)OTL(Port_Data.Port_Write.[Port])OTL(Local_Control.11);
   39: NOP();
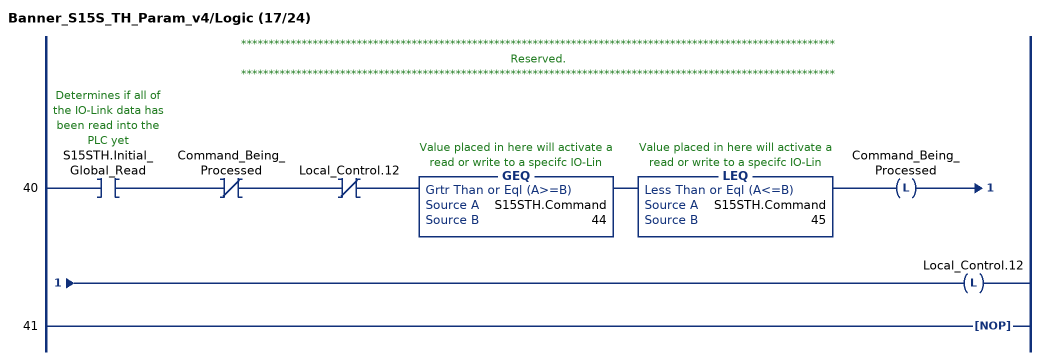
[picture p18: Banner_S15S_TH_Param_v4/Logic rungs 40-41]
   // ************************************************************************************************************
   // Reserved.
   // ************************************************************************************************************
   40: XIC(S15STH.Initial_Global_Read)XIO(Command_Being_Processed)XIO(Local_Control.12)GEQ(S15STH.Command,44)LEQ(S15STH.Command,45)OTL(Command_Being_Processed)OTL(Local_Control.12);
   41: NOP();
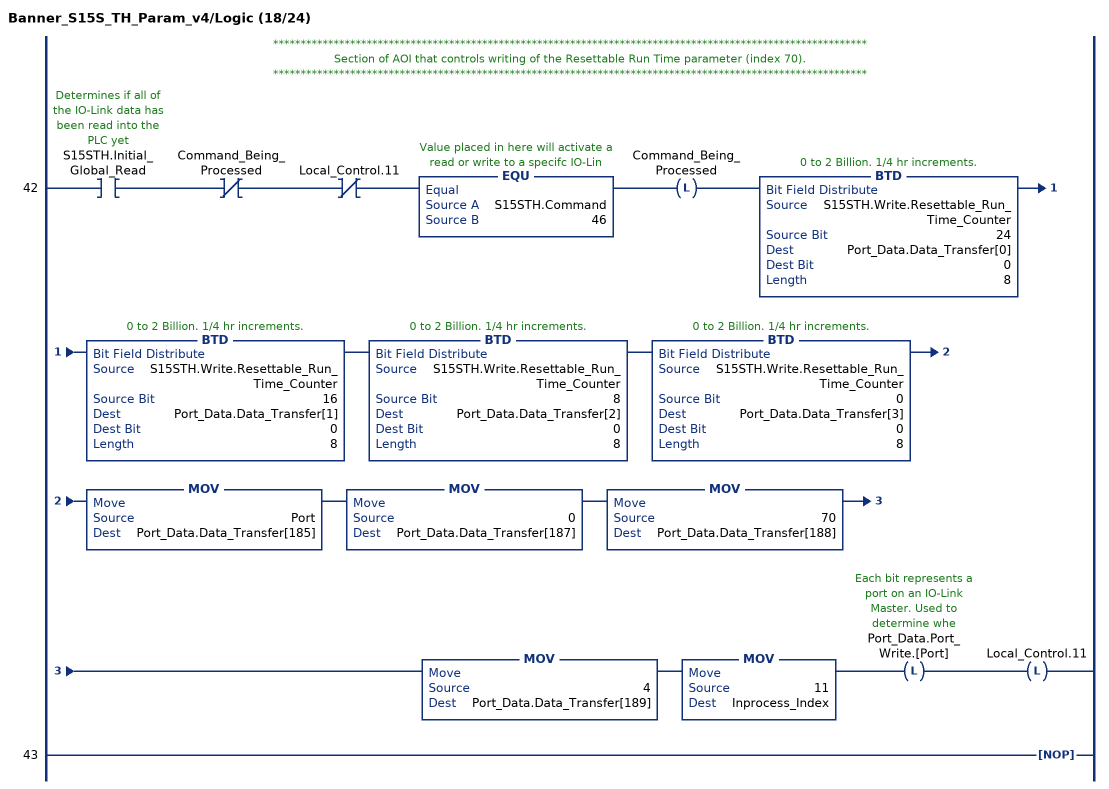
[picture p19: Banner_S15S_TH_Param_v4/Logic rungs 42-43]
   // ************************************************************************************************************
   // Section of AOI that controls writing of the Resettable Run Time parameter (index 70).
   // ************************************************************************************************************
   42: XIC(S15STH.Initial_Global_Read)XIO(Command_Being_Processed)XIO(Local_Control.11)EQU(S15STH.Command,46)OTL(Command_Being_Processed)BTD(S15STH.Write.Resettable_Run_Time_Counter,24,Port_Data.Data_Transfer[0],0,8)BTD(S15STH.Write.Resettable_Run_Time_Counter,16,Port_Data.Data_Transfer[1],0,8)BTD(S15STH.Write.Resettable_Run_Time_Counter,8,Port_Data.Data_Transfer[2],0,8)BTD(S15STH.Write.Resettable_Run_Time_Counter,0,Port_Data.Data_Transfer[3],0,8)MOV(Port,Port_Data.Data_Transfer[185])MOV(0,Port_Data.Data_Transfer[187])MOV(70,Port_Data.Data_Transfer[188])MOV(4,Port_Data.Data_Transfer[189])MOV(11,Inprocess_Index)OTL(Port_Data.Port_Write.[Port])OTL(Local_Control.11);
   43: NOP();
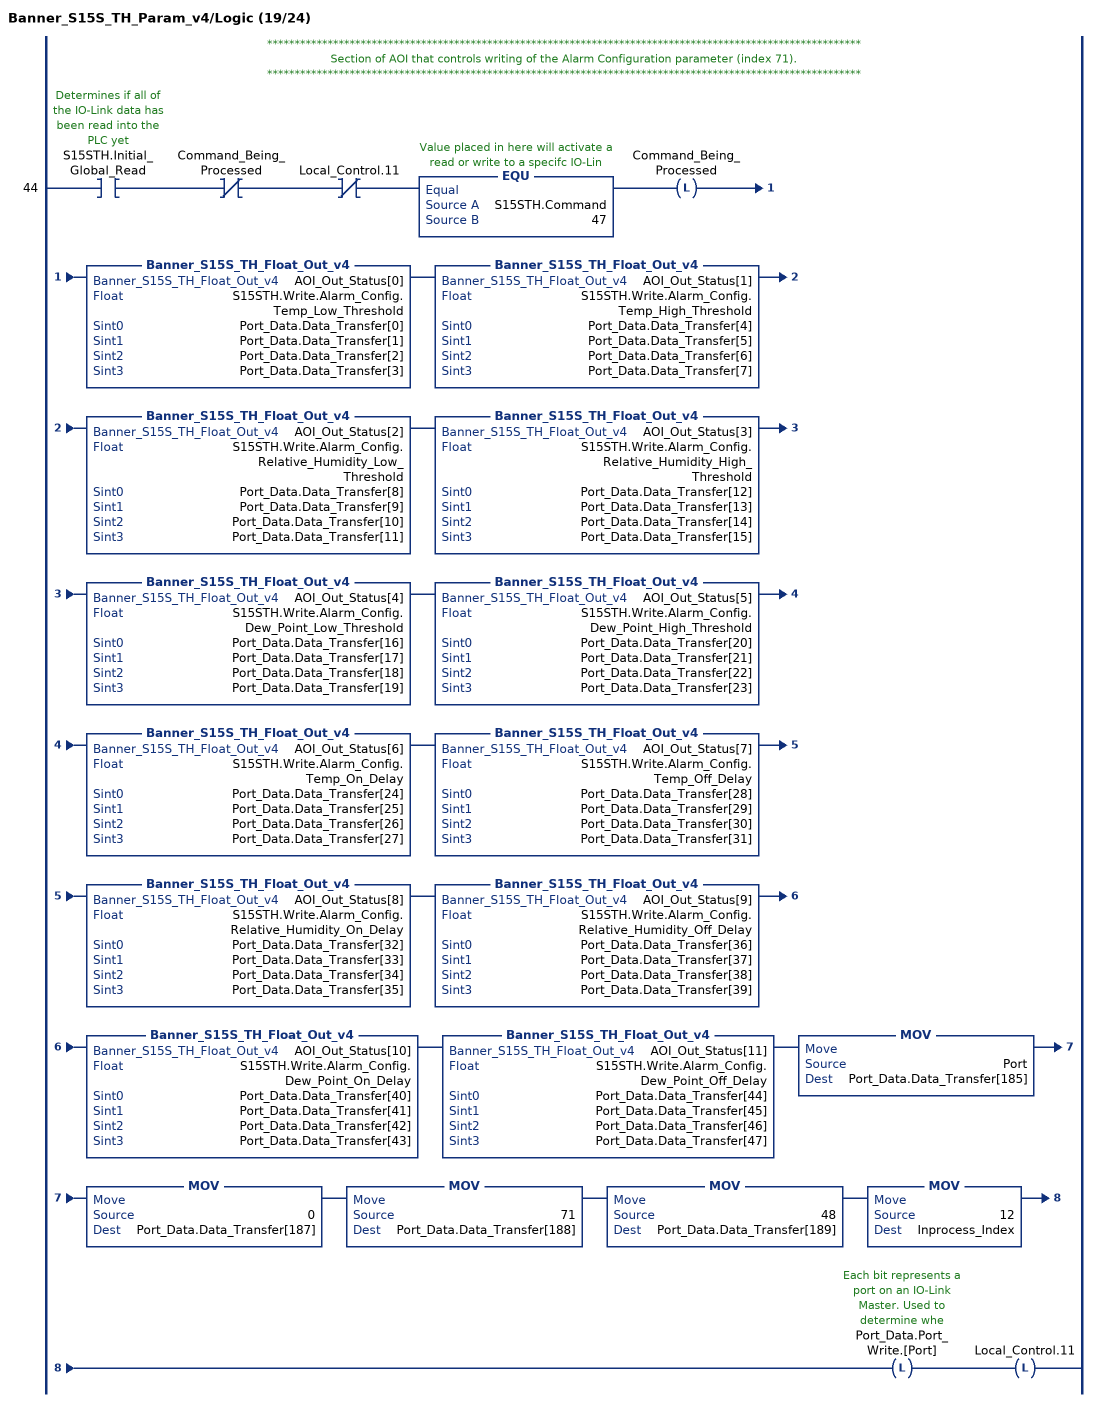
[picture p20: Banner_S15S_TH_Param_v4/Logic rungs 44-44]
   // ************************************************************************************************************
   // Section of AOI that controls writing of the Alarm Configuration parameter (index 71).
   // ************************************************************************************************************
   44: XIC(S15STH.Initial_Global_Read)XIO(Command_Being_Processed)XIO(Local_Control.11)EQU(S15STH.Command,47)OTL(Command_Being_Processed)Banner_S15S_TH_Float_Out_v4(AOI_Out_Status[0],S15STH.Write.Alarm_Config.Temp_Low_Threshold,Port_Data.Data_Transfer[0],Port_Data.Data_Transfer[1],Port_Data.Data_Transfer[2],Port_Data.Data_Transfer[3])Banner_S15S_TH_Float_Out_v4(AOI_Out_Status[1],S15STH.Write.Alarm_Config.Temp_High_Threshold,Port_Data.Data_Transfer[4],Port_Data.Data_Transfer[5],Port_Data.Data_Transfer[6],Port_Data.Data_Transfer[7])Banner_S15S_TH_Float_Out_v4(AOI_Out_Status[2],S15STH.Write.Alarm_Config.Relative_Humidity_Low_Threshold,Port_Data.Data_Transfer[8],Port_Data.Data_Transfer[9],Port_Data.Data_Transfer[10],Port_Data.Data_Transfer[11])Banner_S15S_TH_Float_Out_v4(AOI_Out_Status[3],S15STH.Write.Alarm_Config.Relative_Humidity_High_Threshold,Port_Data.Data_Transfer[12],Port_Data.Data_Transfer[13],Port_Data.Data_Transfer[14],Port_Data.Data_Transfer[15])Banner_S15S_TH_Float_Out_v4(AOI_Out_Status[4],S15STH.Write.Alarm_Config.Dew_Point_Low_Threshold,Port_Data.Data_Transfer[16],Port_Data.Data_Transfer[17],Port_Data.Data_Transfer[18],Port_Data.Data_Transfer[19])Banner_S15S_TH_Float_Out_v4(AOI_Out_Status[5],S15STH.Write.Alarm_Config.Dew_Point_High_Threshold,Port_Data.Data_Transfer[20],Port_Data.Data_Transfer[21],Port_Data.Data_Transfer[22],Port_Data.Data_Transfer[23])Banner_S15S_TH_Float_Out_v4(AOI_Out_Status[6],S15STH.Write.Alarm_Config.Temp_On_Delay,Port_Data.Data_Transfer[24],Port_Data.Data_Transfer[25],Port_Data.Data_Transfer[26],Port_Data.Data_Transfer[27])Banner_S15S_TH_Float_Out_v4(AOI_Out_Status[7],S15STH.Write.Alarm_Config.Temp_Off_Delay,Port_Data.Data_Transfer[28],Port_Data.Data_Transfer[29],Port_Data.Data_Transfer[30],Port_Data.Data_Transfer[31])Banner_S15S_TH_Float_Out_v4(AOI_Out_Status[8],S15STH.Write.Alarm_Config.Relative_Humidity_On_Delay,Port_Data.Data_Transfer[32],Port_Data.Data_Transfer[33],Port_Data.Data_Transfer[34],Port_Data.Data_Transfer[35])Banner_S15S_TH_Float_Out_v4(AOI_Out_Status[9],S15STH.Write.Alarm_Config.Relative_Humidity_Off_Delay,Port_Data.Data_Transfer[36],Port_Data.Data_Transfer[37],Port_Data.Data_Transfer[38],Port_Data.Data_Transfer[39])Banner_S15S_TH_Float_Out_v4(AOI_Out_Status[10],S15STH.Write.Alarm_Config.Dew_Point_On_Delay,Port_Data.Data_Transfer[40],Port_Data.Data_Transfer[41],Port_Data.Data_Transfer[42],Port_Data.Data_Transfer[43])Banner_S15S_TH_Float_Out_v4(AOI_Out_Status[11],S15STH.Write.Alarm_Config.Dew_Point_Off_Delay,Port_Data.Data_Transfer[44],Port_Data.Data_Transfer[45],Port_Data.Data_Transfer[46],Port_Data.Data_Transfer[47])MOV(Port,Port_Data.Data_Transfer[185])MOV(0,Port_Data.Data_Transfer[187])MOV(71,Port_Data.Data_Transfer[188])MOV(48,Port_Data.Data_Transfer[189])MOV(12,Inprocess_Index)OTL(Port_Data.Port_Write.[Port])OTL(Local_Control.11);
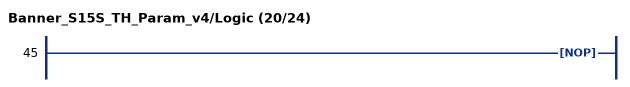
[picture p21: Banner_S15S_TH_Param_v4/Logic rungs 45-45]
   45: NOP();
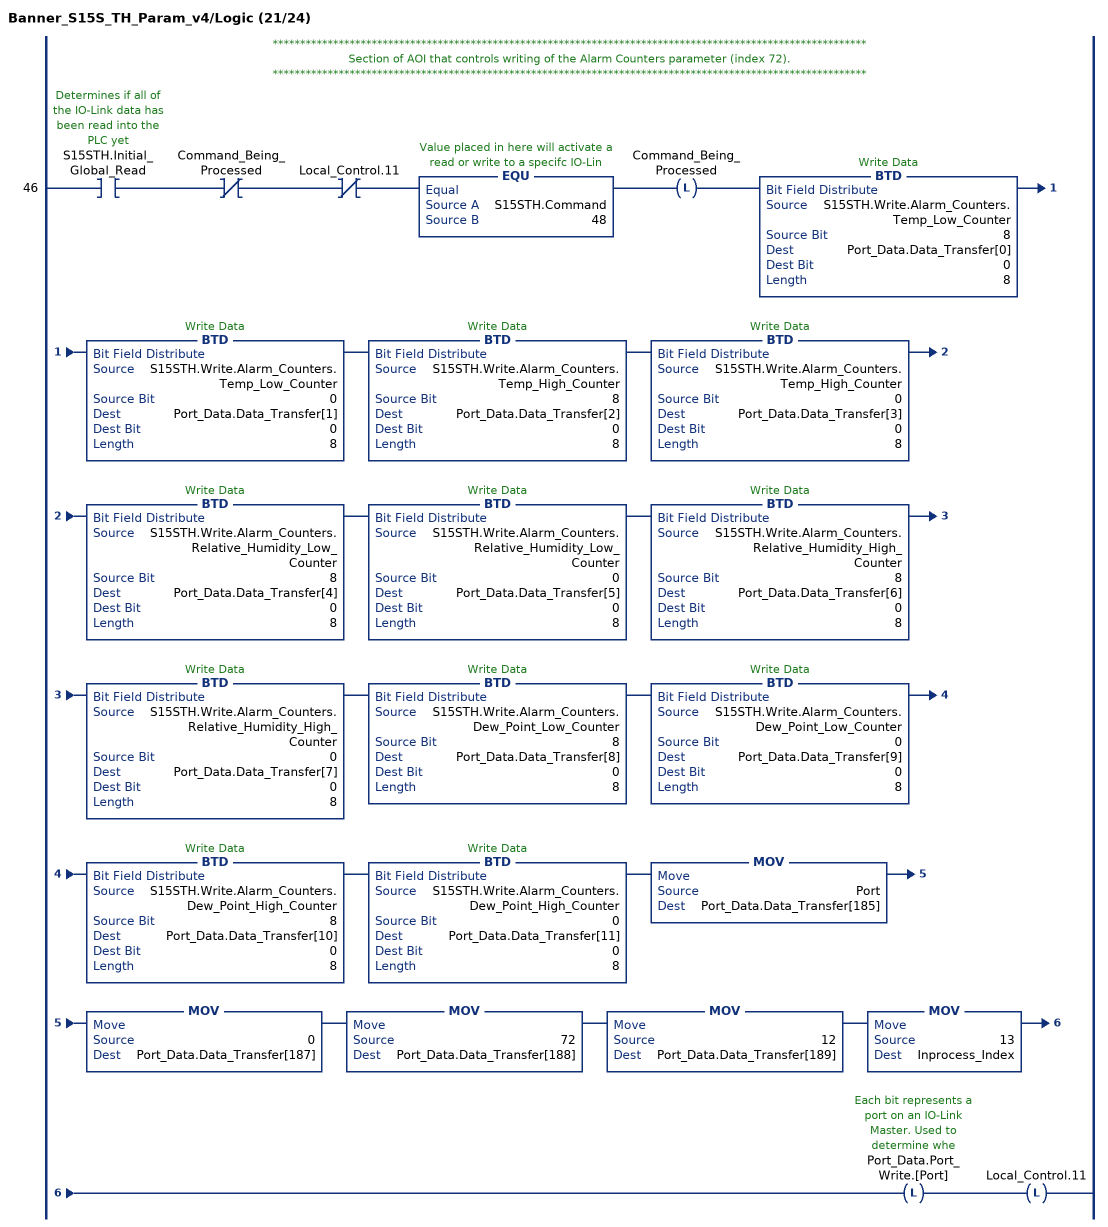
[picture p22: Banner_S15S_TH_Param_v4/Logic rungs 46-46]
   // ************************************************************************************************************
   // Section of AOI that controls writing of the Alarm Counters parameter (index 72).
   // ************************************************************************************************************
   46: XIC(S15STH.Initial_Global_Read)XIO(Command_Being_Processed)XIO(Local_Control.11)EQU(S15STH.Command,48)OTL(Command_Being_Processed)BTD(S15STH.Write.Alarm_Counters.Temp_Low_Counter,8,Port_Data.Data_Transfer[0],0,8)BTD(S15STH.Write.Alarm_Counters.Temp_Low_Counter,0,Port_Data.Data_Transfer[1],0,8)BTD(S15STH.Write.Alarm_Counters.Temp_High_Counter,8,Port_Data.Data_Transfer[2],0,8)BTD(S15STH.Write.Alarm_Counters.Temp_High_Counter,0,Port_Data.Data_Transfer[3],0,8)BTD(S15STH.Write.Alarm_Counters.Relative_Humidity_Low_Counter,8,Port_Data.Data_Transfer[4],0,8)BTD(S15STH.Write.Alarm_Counters.Relative_Humidity_Low_Counter,0,Port_Data.Data_Transfer[5],0,8)BTD(S15STH.Write.Alarm_Counters.Relative_Humidity_High_Counter,8,Port_Data.Data_Transfer[6],0,8)BTD(S15STH.Write.Alarm_Counters.Relative_Humidity_High_Counter,0,Port_Data.Data_Transfer[7],0,8)BTD(S15STH.Write.Alarm_Counters.Dew_Point_Low_Counter,8,Port_Data.Data_Transfer[8],0,8)BTD(S15STH.Write.Alarm_Counters.Dew_Point_Low_Counter,0,Port_Data.Data_Transfer[9],0,8)BTD(S15STH.Write.Alarm_Counters.Dew_Point_High_Counter,8,Port_Data.Data_Transfer[10],0,8)BTD(S15STH.Write.Alarm_Counters.Dew_Point_High_Counter,0,Port_Data.Data_Transfer[11],0,8)MOV(Port,Port_Data.Data_Transfer[185])MOV(0,Port_Data.Data_Transfer[187])MOV(72,Port_Data.Data_Transfer[188])MOV(12,Port_Data.Data_Transfer[189])MOV(13,Inprocess_Index)OTL(Port_Data.Port_Write.[Port])OTL(Local_Control.11);
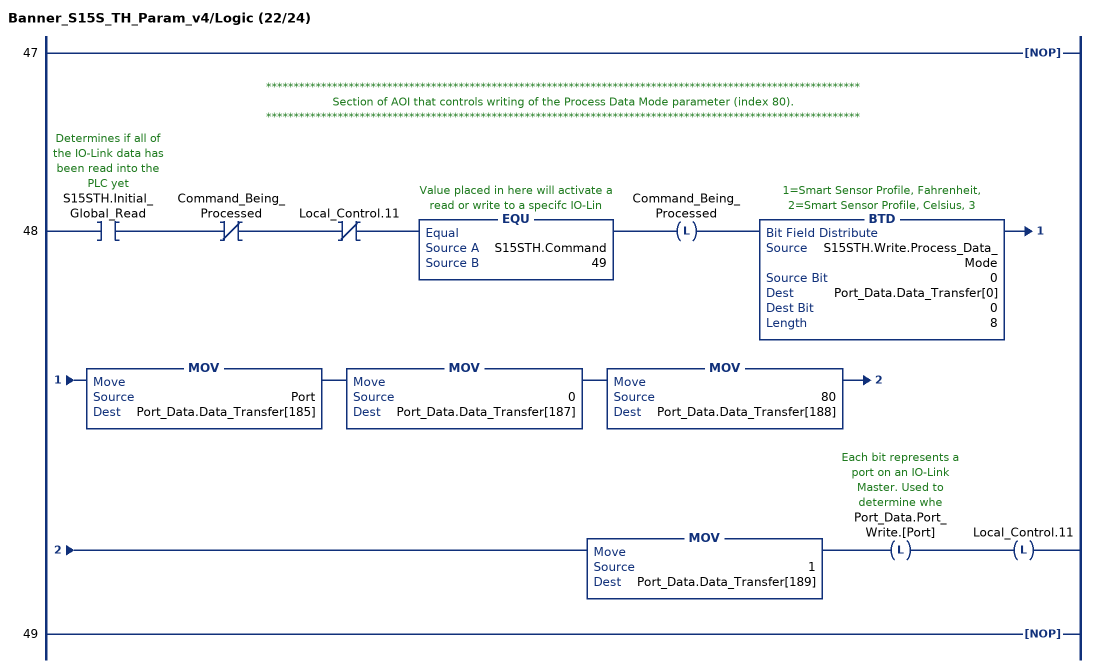
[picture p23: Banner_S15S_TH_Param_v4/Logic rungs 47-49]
   47: NOP();
   // ************************************************************************************************************
   // Section of AOI that controls writing of the Process Data Mode parameter (index 80).
   // ************************************************************************************************************
   48: XIC(S15STH.Initial_Global_Read)XIO(Command_Being_Processed)XIO(Local_Control.11)EQU(S15STH.Command,49)OTL(Command_Being_Processed)BTD(S15STH.Write.Process_Data_Mode,0,Port_Data.Data_Transfer[0],0,8)MOV(Port,Port_Data.Data_Transfer[185])MOV(0,Port_Data.Data_Transfer[187])MOV(80,Port_Data.Data_Transfer[188])MOV(1,Port_Data.Data_Transfer[189])OTL(Port_Data.Port_Write.[Port])OTL(Local_Control.11);
   49: NOP();
